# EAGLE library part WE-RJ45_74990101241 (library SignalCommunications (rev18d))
WE-RJ45 LAN Transformer Order Code 74990101241 Design THT xBase-T 10/100 Base-T Ports 1x1 Application Standard Tab Position Vertical LED (Left-Right) YELLOW-GREEN EMI Fingers No Details see: http://katalog.we-online.de/en/pbs/WE-LAN-RJ45 Created by Yingchun Shan 2016 (C) Wurth Elektronik
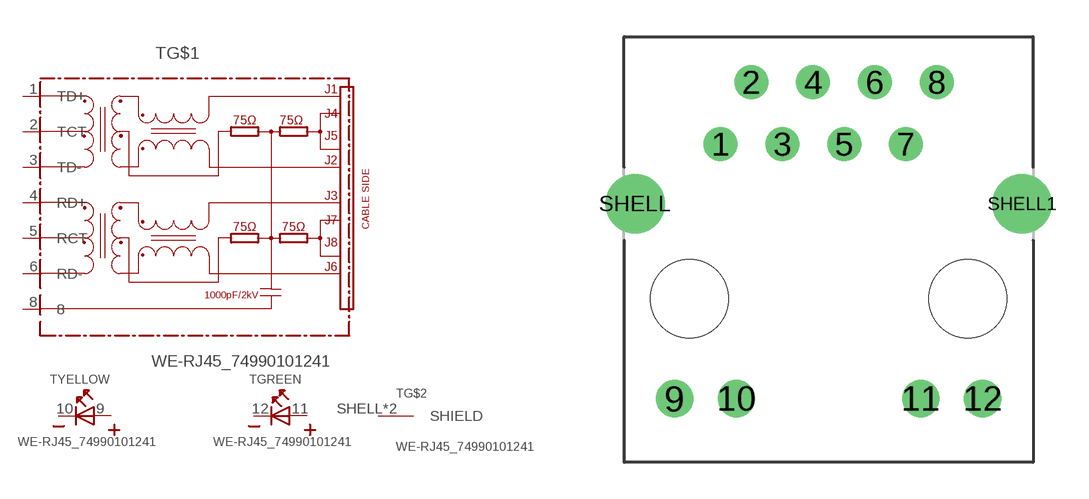
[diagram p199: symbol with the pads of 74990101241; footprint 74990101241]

Designator prefix T; gates G$1=74990101241 YELLOW=LED_2PIN GREEN=LED_2PIN G$2=SHIELD

## WE-RJ45_74990101241  [74990101241]
1  G$1:TD+
2  G$1:TCT
3  G$1:TD-
4  G$1:RD+
5  G$1:RCT
6  G$1:RD-
8  G$1:8
9  YELLOW:A  pas
10  YELLOW:K  pas
11  GREEN:A  pas
12  GREEN:K  pas
SHELL  G$2:SHIELD  pas
SHELL1  G$2:SHIELD  pas

## Footprint 74990101241 (pad centres in mm)
drill 0.89: 1 -4.44,6.35; 2 -3.18,8.89; 3 -1.9,6.35; 4 -0.64,8.89; 5 0.64,6.35; 6 1.9,8.89; 7 3.18,6.35; 8 4.44,8.89
drill 1.02: 9 -6.325,-4.11; 10 -3.785,-4.11; 11 3.785,-4.11; 12 6.325,-4.11
drill 1.63: SHELL -7.95,3.9; SHELL1 7.95,3.9
hole 3.2 at -5.715,0
hole 3.2 at 5.715,0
